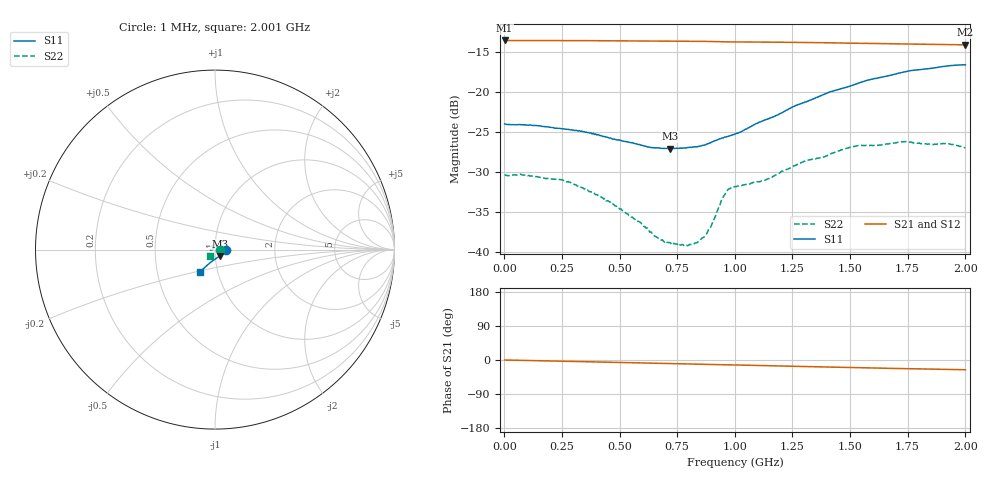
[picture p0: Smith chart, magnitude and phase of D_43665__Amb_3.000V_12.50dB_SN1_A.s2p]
! device id: 43665_
! dir: \\malibu\benchdata\1_engineers\tn_data\43665_75ohm\new\sparar\43665_\amb\3p000v\12p50db
! Serial: 1
! Insertion: A
! Temp: Amb
! VDD: 3.000V
! Attenuation Step: 12.50dB
! IDD: 1.449548e+00mA
! FILE NAME
! DATE 03-27-2009 08:36:26
! CORRECTED  DATA
#  Hz  S  RI  R  75
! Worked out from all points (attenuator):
!   401 points, 1 MHz to 2.001 GHz, reference 75 ohm
!   highest |S21| = -13.58 dB at 1 MHz (marker M1); lowest = -14.1 dB at 2.001 GHz (marker M2)
!   lowest |S11| = -27.1 dB at 721 MHz (marker M3), VSWR 1.09, Z = 78.9 - j5.57 ohm
!   |S11| at or under -10 dB: start of sweep to end of sweep
!   |S22| runs from -39.3 to -26.2 dB; largest |S21 - S12| = 0.0006
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1000000  0.063 -0.000783  0.2094 -0.000258  0.2096 -0.000333  0.0305 -0.000459
2.36e8  0.0584 -0.00954  0.2088 -0.0109  0.2089 -0.0109  0.0266 0.0102
3.36e8  0.055 -0.0143  0.2083 -0.0157  0.2084 -0.0156  0.0214 0.0134
4.61e8  0.0475 -0.0197  0.2076 -0.0216  0.2077 -0.0216  0.0145 0.0144
5.91e8  0.0378 -0.0272  0.2062 -0.0278  0.2062 -0.0277  0.00502 0.0144
6.71e8  0.0312 -0.032  0.2055 -0.0315  0.2055 -0.0315  0.0006 0.0122
7.21e8  0.0267 -0.0352  0.2049 -0.034  0.2049 -0.0339  -0.00223 0.0112
7.91e8  0.0207 -0.0396  0.2039 -0.0376  0.2039 -0.0375  -0.00754 0.00798
8.31e8  0.0167 -0.0422  0.2033 -0.0396  0.2033 -0.0395  -0.0102 0.00514
8.61e8  0.0135 -0.0443  0.2026 -0.0412  0.2026 -0.041  -0.0119 0.0028
9.01e8  0.00892 -0.0478  0.2015 -0.0432  0.2016 -0.043  -0.0149 -0.0007
9.41e8  0.00463 -0.0509  0.2003 -0.0447  0.2004 -0.0444  -0.0206 -0.00296
9.61e8  0.00296 -0.0522  0.1999 -0.0451  0.2 -0.0449  -0.0232 -0.0025
9.81e8  0.00118 -0.0533  0.1997 -0.0456  0.1999 -0.0454  -0.0249 -0.00151
1.001e9  -0.00152 -0.0544  0.1997 -0.0464  0.1998 -0.0462  -0.0256 -0.00137
1.146e9  -0.017 -0.0657  0.1974 -0.0532  0.1977 -0.053  -0.0273 -0.00907
1.336e9  -0.0372 -0.0817  0.1936 -0.0615  0.1939 -0.0614  -0.0316 -0.0211
1.511e9  -0.054 -0.0957  0.1892 -0.0688  0.1896 -0.0688  -0.0334 -0.0309
1.671e9  -0.0665 -0.1076  0.1853 -0.0748  0.1854 -0.0749  -0.032 -0.0349
1.741e9  -0.0714 -0.1128  0.1835 -0.0772  0.1838 -0.0775  -0.0312 -0.0376
1.916e9  -0.08 -0.1204  0.1792 -0.0827  0.1793 -0.0828  -0.0296 -0.0372
2.001e9  -0.0821 -0.1224  0.1772 -0.0853  0.1768 -0.0857  -0.0268 -0.0358
